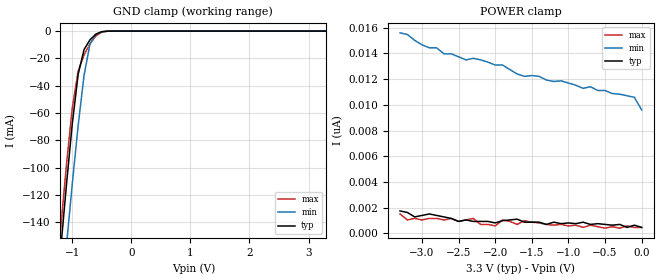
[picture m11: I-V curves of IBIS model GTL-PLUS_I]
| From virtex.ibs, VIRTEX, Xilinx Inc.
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|   Model GTL-PLUS_I
[Model]   GTL-PLUS_I
Model_type   Input
Polarity   Non-Inverting
Vinl =   0.900V
Vinh =   1.100V
C_comp   6.5000pF   5.0000pF   8.0000pF
[Temperature Range]   27.0000   100.0000   0.000
[Voltage Range]   3.3000V   3.0000V   3.6000V
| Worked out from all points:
|   GND clamp passes 1 mA (typ) near -0.53 V on its own axis
[GND_clamp]
| voltage   I(typ)   I(min)   I(max)
-3.3V     -1.286A    -1.272A    -1.289A
-1.2V     -161.8mA   -205.3mA   -146.7mA
-1.1V     -113.2mA   -157.8mA   -98.56mA
-1V       -68.04mA   -112mA     -56.27mA
-900mV    -31.6mA    -69.09mA   -29.2mA
-800mV    -13.5mA    -32.35mA   -17.42mA
-700mV    -6.408mA   -9.456mA   -9.303mA
-600mV    -2.237mA   -2.349mA   -3.538mA
-500mV    -423.5uA   -545.4uA   -698.2uA
-400mV    -42.44uA   -91.29uA   -59.93uA
3.3V      465.7pA    42.32nA    407.5pA
[POWER_clamp]
| voltage   I(typ)   I(min)   I(max)
-3.3V     1.746nA    15.6nA     1.513nA
-3.2V     1.63nA     15.48nA    1.048nA
-3.1V     1.281nA    15.02nA    1.164nA
-2.7V     1.281nA    13.97nA    1.048nA
-2.3V     931.3pA    13.62nA    1.164nA
-2.2V     931.3pA    13.5nA     698.5pA
-2V       814.9pA    13.1nA     582.1pA
-1.9V     989.5pA    13.1nA     1.048nA
-1.7V     1.106nA    12.4nA     698.5pA
-1.6V     873.1pA    12.22nA    989.5pA
-100mV    640.3pA    10.59nA    465.7pA
0V        465.7pA    9.604nA    465.7pA
